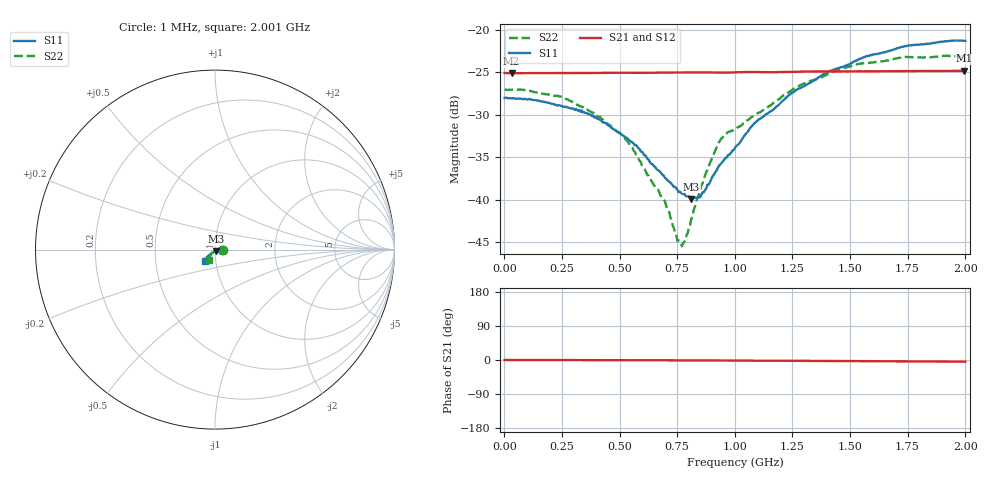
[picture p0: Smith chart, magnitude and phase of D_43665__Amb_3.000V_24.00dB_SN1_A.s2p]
! device id: 43665_
! dir: \\malibu\benchdata\1_engineers\tn_data\43665_75ohm\new\sparar\43665_\amb\3p000v\24p00db
! Serial: 1
! Insertion: A
! Temp: Amb
! VDD: 3.000V
! Attenuation Step: 24.00dB
! IDD: 1.445997e+00mA
! FILE NAME
! DATE 03-27-2009 08:39:16
! CORRECTED  DATA
#  Hz  S  RI  R  75
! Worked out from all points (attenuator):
!   401 points, 1 MHz to 2.001 GHz, reference 75 ohm
!   highest |S21| = -24.84 dB at 1.996 GHz (marker M1); lowest = -25.1 dB at 31 MHz (marker M2)
!   lowest |S11| = -39.9 dB at 811 MHz (marker M3), VSWR 1.02, Z = 75.6 - j1.4 ohm
!   |S11| at or under -10 dB: start of sweep to end of sweep
!   |S22| runs from -45.5 to -23.1 dB; largest |S21 - S12| = 0.00031
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1000000  0.0396 -0.000431  0.0556 -0.00017  0.0557 -3.26e-05  0.0446 -0.000328
3.1e7  0.0394 -0.000146  0.0554 -4.11e-05  0.0555 -3.02e-05  0.0444 0.000444
2.36e8  0.0359 -0.000346  0.0556 -0.000149  0.0556 -0.000145  0.0402 0.00555
3.36e8  0.0335 -0.00108  0.0556 -0.000278  0.0556 -0.000248  0.0345 0.00677
4.16e8  0.0294 -0.00116  0.0557 -0.00031  0.0557 -0.000265  0.03 0.00646
5.26e8  0.0231 -0.00258  0.0558 -0.000568  0.0558 -0.000477  0.0222 0.0044
6.71e8  0.0136 -0.00572  0.0558 -0.000728  0.0559 -0.00063  0.0112 -2.16e-05
7.06e8  0.0113 -0.0066  0.0559 -0.000791  0.0559 -0.000708  0.00878 -0.00118
7.61e8  0.0076 -0.00815  0.0559 -0.000953  0.056 -0.000835  0.00421 -0.00363
7.81e8  0.00633 -0.00877  0.056 -0.00104  0.056 -0.000894  0.00227 -0.00518
8.11e8  0.00401 -0.00925  0.056 -0.00111  0.056 -0.000989  1.82e-05 -0.00769
8.56e8  0.000293 -0.0107  0.056 -0.00127  0.0561 -0.00113  -0.00331 -0.0118
9.26e8  -0.00582 -0.0142  0.0559 -0.00149  0.056 -0.00132  -0.0106 -0.0181
9.61e8  -0.00808 -0.0157  0.0558 -0.0014  0.0559 -0.00122  -0.0161 -0.0183
1.001e9  -0.0114 -0.0166  0.056 -0.00132  0.0561 -0.00118  -0.0189 -0.0178
1.096e9  -0.0198 -0.0211  0.0562 -0.00194  0.0563 -0.00174  -0.0211 -0.024
1.241e9  -0.0305 -0.0284  0.0564 -0.00201  0.0565 -0.00182  -0.0261 -0.0347
1.336e9  -0.0362 -0.0339  0.0567 -0.00236  0.0568 -0.00216  -0.0291 -0.041
1.526e9  -0.0475 -0.0454  0.0568 -0.00309  0.0569 -0.00298  -0.0335 -0.0526
1.671e9  -0.0524 -0.0537  0.0569 -0.00359  0.057 -0.00348  -0.0338 -0.057
1.996e9  -0.0552 -0.0658  0.0571 -0.00439  0.0572 -0.00442  -0.0321 -0.0609
2.001e9  -0.0555 -0.0657  0.0571 -0.00439  0.0571 -0.0044  -0.0322 -0.0606
